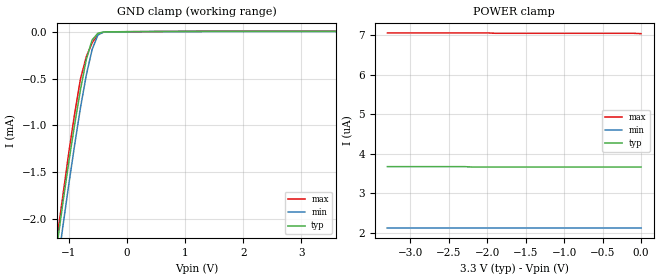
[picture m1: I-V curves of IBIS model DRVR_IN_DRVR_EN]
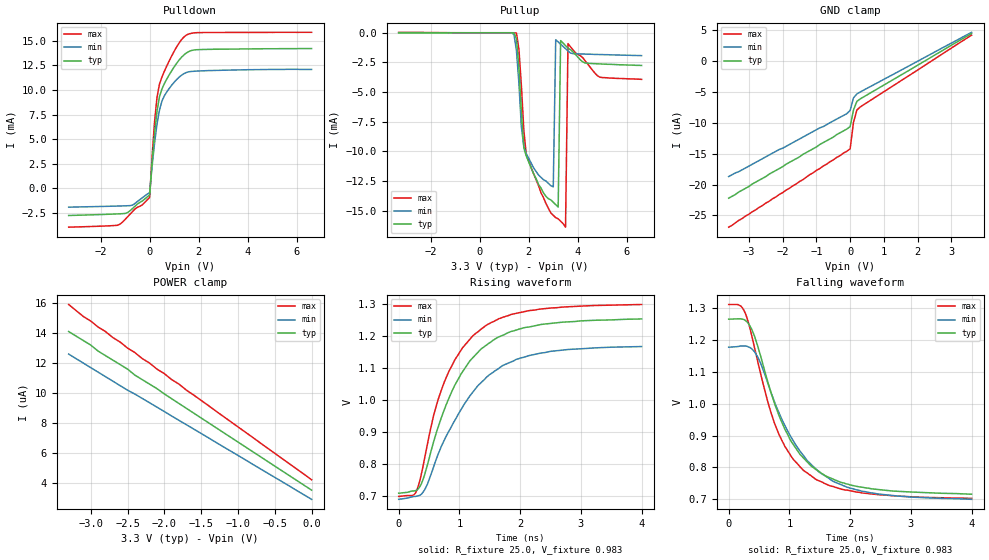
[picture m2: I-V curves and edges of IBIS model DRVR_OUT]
|   Texas Instruments Incorporated
|   Data Transmissions Products
|   IBIS Model for SN65MLVD128
|   48DGG TSSOP Package
[IBIS Ver]   3.2
[Comment char]   |_char
[File name]   mlvd128.ibs
[File Rev]   1.0
[Date]   31Jan04
[Source]   File originated at Texas Instruments Incorporated.
   Data Transmission Products Group. All data based on
   Simulation Measurements.
[Notes]
[Disclaimer]
(C) Copyright Texas Instruments Incorporated 2004
   All rights reserved
  Texas Instruments Incorporated hereby grants the user of this IBIS
model a non-exclusive, nontransferable license to use this IBIS model
under the following terms.  Before using this IBIS model, the user
should read this license.  If the user does not accept these terms,
the IBIS model should be returned to Texas Instruments within 30 days.
  The user is granted this license only to use the IBIS model and
is not granted rights to sell, load, rent, lease or license the IBIS
model in whole or in part, or in modified form to anyone other than
user.  User may modify the IBIS model to suit its specific applications
but rights to derivative works and such modifications shall belong to
Texas Instruments.
  This IBIS model is provided on an "AS IS" basis and Texas Instruments
makes absolutely no warranty with respect to the information contained
herein.  TEXAS INSTRUMENTS DISCLAIMS AND CUSTOMER WAIVES ALL WARRANTIES,
EXPRESS OR IMPLIED, INCLUDING WARRANTIES OF MERCHANTABILITY OR FITNESS
FOR A PARTICULAR PURPOSE. The entire risk as to quality and performance
is with the Customer. ACCORDINGLY, IN NO EVENT SHALL THE COMPANY BE LIABLE
FOR ANY DAMAGES, WHETHER IN CONTRACT OR TORT,INCLUDING ANY LOST PROFITS
OR OTHER INCIDENTAL, CONSEQUENTIAL, EXEMPLARY, OR PUNITIVE DAMAGES ARISING
OUT OF THE USE OR APPLICATION OF THE IBIS model provided in this package.
Further, Texas Instruments reserves the right to discontinue or make changes
without notice to any product herein to improve reliability, function, or
design. Texas Instruments does not convey any license under patent rights
or any other intellectual property rights, including those of third parties.
Contact Texas Instruments at ATTN:DATA TRANSMISSIONS
[Copyright]   Copyright 2004, Texas Instruments, All Rights Reserved
[Component]   SN65MLVD128DGG
[Manufacturer]  Texas Instruments Incorporated
[Package]
|   typ   min   max
R_pkg   0.044   0.038   0.051
L_pkg   3.019nH   2.486nH   4.099nH
C_pkg   0.507pF   0.334pF   0.809pF
[Pin]   signal_name   model_name   R_pin   L_pin   C_pin
1   VCC   POWER   0.041   4.017n   0.759p
2   1A   DRVR_OUT   0.042   3.737n   0.792p
3   1B   DRVR_OUT   0.042   3.48n   0.661p
4   2A   DRVR_OUT   0.038   3.131n   0.575p
5   2B   DRVR_OUT   0.047   3.122n   0.566p
6   GND   GND   0.043   2.948n   0.504p
7   VCC   POWER   0.045   2.845n   0.397p
8   3A   DRVR_OUT   0.049   2.835n   0.394p
9   3B   DRVR_OUT   0.048   2.715n   0.378p
10   4A   DRVR_OUT   0.05   2.664n   0.363p
11   4B   DRVR_OUT   0.05   2.585n   0.348p
12   GND   GND   0.049   2.55n   0.337p
13   VCC   POWER   0.049   2.541n   0.336p
14   5A   DRVR_OUT   0.05   2.574n   0.348p
15   5B   DRVR_OUT   0.049   2.618n   0.359p
16   6A   DRVR_OUT   0.046   2.671n   0.375p
17   6B   DRVR_OUT   0.045   2.754n   0.389p
18   GND   GND   0.044   2.823n   0.450p
19   VCC   POWER   0.042   2.968n   0.503p
20   7A   DRVR_OUT   0.051   3.108n   0.535p
21   7B   DRVR_OUT   0.042   3.175n   0.587p
22   8A   DRVR_OUT   0.041   3.449n   0.678p
23   8B   DRVR_OUT   0.044   3.766n   0.804p
24   GND   GND   0.043   4.065n   0.761p
25   GND   GND   0.041   3.994n   0.757p
26   GND   GND   0.039   3.649n   0.789p
27   EN8   DRVR_IN_DRVR_EN  0.038   3.362n   0.660p
28   EN7   DRVR_IN_DRVR_EN  0.038   3.082n   0.574p
29   VCC   POWER   0.044   2.99n   0.522p
30   VCC   POWER   0.041   2.917n   0.495p
31   GND   GND   0.043   2.82n   0.448p
32   EN6   DRVR_IN_DRVR_EN  0.043   2.699n   0.385p
33   EN5   DRVR_IN_DRVR_EN  0.045   2.628n   0.372p
34   NC   NC   0.046   2.556n   0.356p
35   VCC   POWER   0.046   2.495n   0.344p
36   VCC   POWER   0.047   2.487n   0.334p
37   GND   GND   0.047   2.49n   0.335p
38   GND   GND   0.046   2.486n   0.343p
39   1D   DRVR_IN_DRVR_EN  0.045   2.566n   0.356p
40   EN4   DRVR_IN_DRVR_EN  0.044   2.639n   0.374p
41   EN3   DRVR_IN_DRVR_EN  0.043   2.701n   0.386p
42   NC   NC   0.043   2.817n   0.450p
43   GND   GND   0.041   2.935n   0.501p
44   GND   GND   0.047   3.035n   0.529p
45   EN2   DRVR_IN_DRVR_EN  0.043   3.171n   0.589p
46   EN1   DRVR_IN_DRVR_EN  0.04   3.415n   0.682p
47   VCC   POWER   0.043   3.741n   0.809p
48   VCC   POWER   0.044   4.099n   0.764p
| Models and submodels in the file (2): DRVR_IN_DRVR_EN (Input), DRVR_OUT (Output)
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|   Driver/Driver Enable Model
[Model]   DRVR_IN_DRVR_EN
Model_type   Input
|Signals   1D, EN1 thru EN8
Vinh = 2.0
Vinl = 0.8
|   typ   min   max
C_comp   4.04pF   3.87pF   4.24pF
|   typ   min   max
[Temperature Range]   25.0   85   -40
[Voltage range]   3.3V   3.0V   3.6V
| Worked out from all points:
|   GND clamp passes 1 mA (typ) near -0.90 V on its own axis
[GND_clamp]
|   Voltage   I(typ)   I(min)   I(max)
-3.6V     -16.3mA    -15.9mA    -16.8mA
-1.2V     -2.27mA    -2.53mA    -2.19mA
-1.1V     -1.82mA    -2.07mA    -1.74mA
-1V       -1.39mA    -1.63mA    -1.29mA
-900mV    -992uA     -1.21mA    -876uA
-800mV    -621uA     -813uA     -505uA
-700mV    -299uA     -466uA     -268uA
-600mV    -88.7uA    -191uA     -120uA
-500mV    -15.9uA    -35.6uA    -26.5uA
-400mV    -2.37uA    -3.13uA    -3.62uA
-300mV    -1.1uA     -793nA     -1.87uA
3.6V      3.66uA     2.11uA     7.04uA
[Power_clamp]
| Note that the[POWER_clamp]voltage table is referenced to Vcc
| and is calculated using Vtable=Vcc - Vmeasured.
|   Voltage   I(typ)   I(min)   I(max)
-3.3V     3.67uA     2.11uA     7.06uA
-2.3V     3.67uA     2.11uA     7.06uA
-2.2V     3.66uA     2.11uA     7.06uA
-2V       3.66uA     2.11uA     7.06uA
-1.9V     3.66uA     2.11uA     7.05uA
-100mV    3.66uA     2.11uA     7.05uA
0V        3.66uA     2.11uA     7.04uA
|   Driver Output/Receiver Input Model
[Model]   DRVR_OUT
Model_type   Output
| Signals   1A through 8A, 1B through 8B
Vmeas = 1.0V   |Reference voltage for timing measurements
Cref = 3pF   |Timing specification test load capacitance value
| variable   typ   min   max
C_comp   3.93pF   3.71pF   4.23pF
|   typ   min   max
[Temperature Range]   25.0   85   -40
[Voltage range]   3.3V   3.0V   3.6V
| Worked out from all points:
|   slope of the pulldown table from 0 to 0.495 V, typ, clamps not added: 46.2 ohm
|   rising waveform, R_fixture 25.0, V_fixture 0.983: 20-80 % time 780ps typ, 884ps min, 694ps max; typ from 0.709 V to 1.25 V
|   falling waveform, R_fixture 25.0, V_fixture 0.983: 20-80 % time 734ps typ, 822ps min, 659ps max; typ from 1.26 V to 0.716 V
[Pulldown]
|   Voltage   I(typ)   I(min)   I(max)
-3.3V     -2.76mA    -1.912mA   -3.946mA
-1.3V     -2.598mA   -1.8mA     -3.75mA
-700mV    -2.055mA   -1.706mA   -2.366mA
0V        -661.3uA   -444.3uA   -917.6uA
100mV     2.646mA    2.245mA    3.252mA
200mV     5.55mA     4.605mA    6.771mA
300mV     7.851mA    6.536mA    9.257mA
400mV     9.314mA    7.951mA    10.59mA
700mV     11.12mA    9.812mA    12.45mA
1.4V      13.57mA    11.66mA    15.39mA
1.9V      14.09mA    11.92mA    15.82mA
6.6V      14.21mA    12.09mA    15.86mA
[Pullup]
|   Voltage   I(typ)   I(min)   I(max)
| Note that the[Pullup]voltage table is referenced to Vcc
| and is calculated using Vtable=Vcc - Vmeasured.
-3.3V     768nA      50nA       36.2uA
1.5V      -514uA     -1.5mA     -22.1uA
1.8V      -9.71mA    -9.57mA    -8.22mA
1.9V      -10.4mA    -10.2mA    -10.3mA
3V        -14.3mA    -13mA      -15.4mA
3.1V      -14.5mA    -590uA     -15.6mA
3.2V      -14.7mA    -775uA     -15.7mA
3.3V      -661uA     -965uA     -15.9mA
3.5V      -1.09mA    -1.34mA    -16.4mA
3.6V      -1.29mA    -1.54mA    -918uA
4.9V      -2.63mA    -1.84mA    -3.75mA
6.6V      -2.76mA    -1.93mA    -3.93mA
[GND_clamp]
|   Voltage   I(typ)   I(min)   I(max)
| Outputs in High Impedance (off)
-3.6V     -22.2uA    -18.7uA    -26.9uA
-800mV    -13.2uA    -10.6uA    -17uA
-100mV    -11uA      -8.51uA    -14.6uA
0V        -10.6uA    -7.97uA    -14.2uA
100mV     -7.89uA    -5.93uA    -9.89uA
200mV     -6.51uA    -5.3uA     -7.91uA
400mV     -5.78uA    -4.68uA    -7.05uA
3.6V      4.51uA     4.69uA     4.24uA
[Power_clamp]
| Note that the[POWER_clamp]voltage table is referenced to Vcc
| and is calculated using Vtable=Vcc - Vmeasured.
|   Voltage   I(typ)   I(min)   I(max)
-3.3V     14.1uA     12.6uA     15.9uA
-3.1V     13.5uA     12uA       15.1uA
-3V       13.2uA     11.7uA     14.8uA
-2.9V     12.8uA     11.4uA     14.4uA
-2.8V     12.5uA     11.1uA     14.1uA
-2.5V     11.6uA     10.2uA     13uA
-2.4V     11.2uA     9.94uA     12.7uA
-2.1V     10.3uA     9.07uA     11.6uA
-1.8V     9.31uA     8.19uA     10.6uA
-1.7V     8.99uA     7.9uA      10.2uA
0V        3.55uA     2.94uA     4.24uA
[Ramp]
|   typ   min   max
dV/dt_r   334mV/819ps   292mV/930ps   369mV/724ps
dV/dt_f   334mV/774ps   292mV/866ps   369mV/702ps
R_load = 25ohm  | Note: The measurement is single-ended with 25ohm
|   to common mode voltage.
[Rising Waveform]
R_fixture = 25.0
V_fixture = 0.983
V_fixture_min = 0.928
V_fixture_max = 0.999
C_fixture = 0p
L_fixture = 0n
|   V(typ)   V(min)   V(max)
0s        709mV      690mV      699mV
275ps     717mV      699mV      709mV
350ps     730mV      703mV      749mV
450ps     782mV      728mV      840mV
575ps     869mV      791mV      951mV
750ps     969mV      874mV      1.055V
1.025ns   1.08V      969mV      1.154V
1.375ns   1.161V     1.057V     1.223V
2.15ns    1.227V     1.138V     1.278V
4ns       1.252V     1.166V     1.297V
[Falling Waveform]
R_fixture = 25.0
V_fixture = 0.983
V_fixture_min = 0.928
V_fixture_max = 0.999
C_fixture = 0p
L_fixture = 0n
|   V(typ)   V(min)   V(max)
0s        1.265V     1.177V     1.311V
225ps     1.265V     1.181V     1.301V
425ps     1.212V     1.163V     1.176V
650ps     1.064V     1.061V     1.002V
825ps     965mV      973mV      905mV
1.025ns   883mV      896mV      836mV
1.25ns    826mV      833mV      788mV
1.725ns   763mV      756mV      740mV
2.2ns     738mV      725mV      720mV
4ns       716mV      700mV      703mV
